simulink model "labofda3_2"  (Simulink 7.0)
settings: Solver=ode45  SolverMode=SingleTasking  StartTime=0.0  StopTime=3  FixedStep=0.05  RelTol=1e-3  AbsTol=1e-6
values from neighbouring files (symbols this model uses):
  L = tf(100,conv([1 2 1],[0.01 1]))    [labofda3.m]
  R = 2    [labofda3.m]

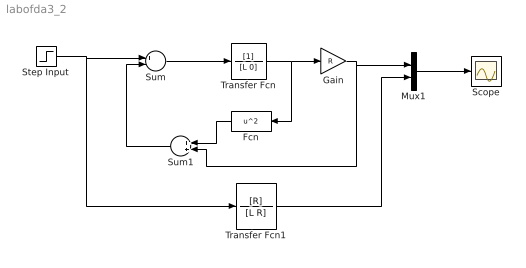
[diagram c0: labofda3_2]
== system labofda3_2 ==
  Fcn : Fcn  Orientation=left  Expr=u^2
  Gain : Gain  Gain=R
  Mux1 : Mux  Inputs=2
  Scope : Scope
  Step Input : Step  Time=0
  Sum : Sum  Inputs=+-
  Sum1 : Sum  Orientation=left
  Transfer Fcn : TransferFcn  Denominator=[L 0]
  Transfer Fcn1 : TransferFcn  Numerator=[R]  Denominator=[L R]
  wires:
  Sum/1 -> Transfer Fcn/1
  Mux1/1 -> Scope/1
  Transfer Fcn/1 -> Gain/1, Fcn/1
  Fcn/1 -> Sum1/1
  Sum1/1 -> Sum/2
  Step Input/1 -> Sum/1, Transfer Fcn1/1
  Gain/1 -> Sum1/2, Mux1/1
  Transfer Fcn1/1 -> Mux1/2
